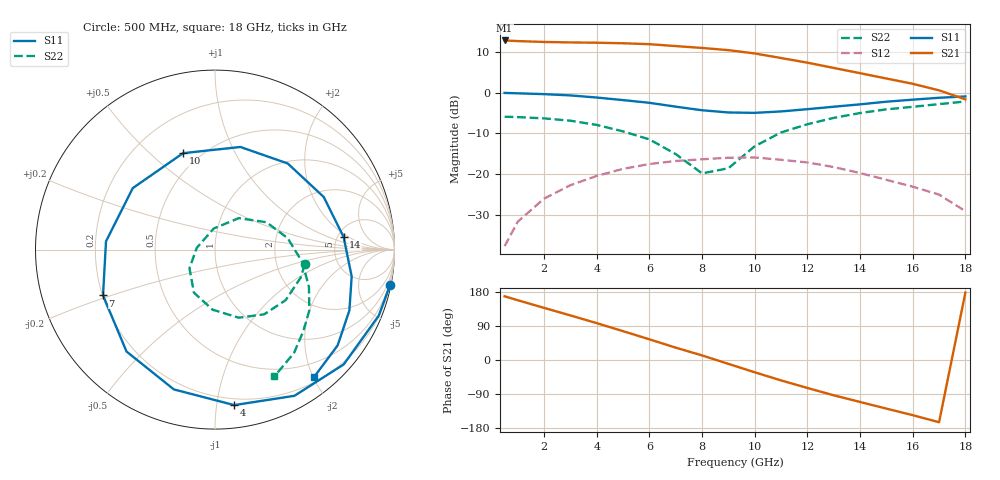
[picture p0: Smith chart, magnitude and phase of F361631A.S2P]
!ATF-36163
!1.5V 10mA
! last updated 11-10-95
# ghz s ma r 50
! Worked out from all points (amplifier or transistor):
!   19 points, 500 MHz to 18 GHz, reference 50 ohm
!   highest |S21| = 12.9 dB at 500 MHz (marker M1)
!   |S21| within 3 dB of that: start of sweep to 9.759 GHz
!   unconditionally stable (mu >= 1): 11.1 GHz to end of sweep
!   at 3 GHz: K = 0.32, MSG = 17.6 dB, |S12| = -22.7 dB
!   at 9 GHz: K = 0.85, MSG = 13.2 dB, |S12| = -16.0 dB
!   at 18 GHz: K = 1.80, MAG = 8.6 dB, |S12| = -29.1 dB
!   lowest NFmin = 0.48 dB at 2 GHz
!   S11 on the Smith chart (normalised r, x): 500 MHz: 0, -10; 4 GHz: 0.15, -1.12; 7 GHz: 0.20, -0.19; 10 GHz: 0.41, +0.64; 14 GHz: 5.65, +1.65; 18 GHz: 0.27, -2.01
0.5  0.995 -11.3  4.392 168.1  0.013 79.3  0.507 -9.3
1  0.984 -21.9  4.314 157.7  0.026 71.2  0.502 -18.3
2  0.961 -41.7  4.208 137.5  0.05 55.5  0.484 -35.6
3  0.927 -61.5  4.154 117.6  0.073 39.8  0.453 -52.7
4  0.873 -82.9  4.119 97.3  0.095 23.2  0.402 -70.8
5  0.812 -106.4  4.057 76.0  0.116 5.6  0.335 -92.3
6  0.752 -131.0  3.952 54.5  0.133 -11.8  0.267 -116.1
7  0.674 -157.8  3.746 32.6  0.145 -30.2  0.176 -143.9
8  0.609 175.7  3.552 12.1  0.152 -44.6  0.102 174.4
9  0.572 143.2  3.338 -10.2  0.159 -60.7  0.118 93.3
10  0.566 108.3  3.04 -32.4  0.16 -77.1  0.22 52.9
11  0.589 76.1  2.671 -53.9  0.15 -92.6  0.325 28.0
12  0.628 49.8  2.342 -73.8  0.139 -106.0  0.41 8.9
13  0.673 25.8  2.018 -93.2  0.122 -119.3  0.491 -8.1
14  0.72 5.6  1.74 -110.7  0.103 -128.9  0.563 -21.6
15  0.776 -11.1  1.495 -128.3  0.085 -138.1  0.625 -32.8
16  0.822 -24.4  1.288 -145.6  0.07 -143.8  0.671 -42.9
17  0.867 -38.0  1.07 -164.2  0.056 -151.4  0.725 -52.7
18  0.9 -52.3  0.829 178.0  0.035 -159.3  0.78 -64.9
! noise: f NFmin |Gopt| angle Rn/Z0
2  0.48  0.781  27.94  0.377
3  0.53  0.747  41.27  0.317
5  0.61  0.604  71.45  0.199
7  0.71  0.477  104.7  0.116
9  0.83  0.322  137.8  0.074
10  0.89  0.232  169.6  0.07
12  1.05  0.195  -92.38  0.126
14  1.24  0.357  -16.44  0.317
16  1.51  0.594  18.91  0.602
18  1.89  0.699  50.92  1.153
